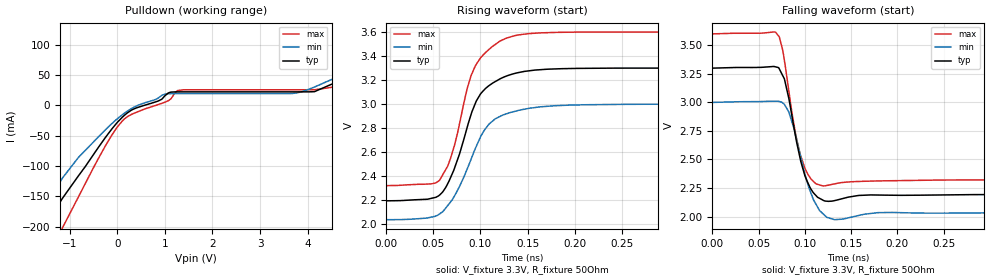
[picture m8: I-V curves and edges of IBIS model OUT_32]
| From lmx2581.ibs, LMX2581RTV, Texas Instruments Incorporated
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[Model]   OUT_32
Model_type   Open_drain
Polarity   Non-Inverting
Vmeas = 3.3
Vref = 3.3
Cref = 1pF
Rref = 50
|   typ   min   max
|   (nom PVT)   (slow PVT)   (fast PVT)
C_comp   0.269p   0.254p   0.289p
|C_comp (Hi state)   0.335p   0.327p   0.337p
|C_comp (Low state)   0.269p   0.254p   0.289p
[Voltage Range]   3.3   3   3.6
[Temperature Range]   27   125   -40
[Pullup Reference]   3.3   3   3.6
[Pulldown Reference]   0   0   0
[Power Clamp Reference]   3.3   3   3.6
[GND Clamp Reference]   0   0   0
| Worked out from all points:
|   slope of the pulldown table from 0 to 0.495 V, typ, clamps not added: 18.7 ohm
|   falling waveform, V_fixture 3.3V, R_fixture 50Ohm: 20-80 % time 16.5ps typ, 18.6ps min, 15.7ps max; typ from 3.3 V to 2.19 V
|   rising waveform, V_fixture 3.3V, R_fixture 50Ohm: 20-80 % time 29.8ps typ, 34.5ps min, 27.4ps max; typ from 2.19 V to 3.3 V
[Pulldown]
|   Voltage   I(typ)   I(min)   I(max)
-3.3V     -460.2mA   -399.9mA   -604.6mA
-2.122V   -291mA     -253.2mA   -382.1mA
-1.3V     -172.4mA   -139.2mA   -229.3mA
-1.152V   -153.4mA   -120.1mA   -202.1mA
16.5mV    -26.96mA   -21.26mA   -34.35mA
293.7mV   -8.221mA   -5.668mA   -15.28mA
986.7mV   14.45mA    18.01mA    4.661mA
1.403V    22.09mA    19.23mA    25.53mA
3.67V     22.1mA     19.42mA    25.56mA
4.145V    22.52mA    30.13mA    25.58mA
4.729V    42.4mA     50.37mA    32.14mA
6.6V      128mA      123.1mA    128.5mA
[Ramp]
R_load = 50
|   typ   min   max
dV/dt_r   0.662764/2.98253e-11   0.576799/3.45445e-11   0.766967/2.7376e-11
dV/dt_f   0.662835/1.65323e-11   0.576841/1.85913e-11   0.767074/1.56776e-11
[Falling Waveform]
V_fixture = 3.3V
V_fixture_min = 3V
V_fixture_max = 3.6V
R_fixture = 50Ohm
C_fixture = 0F
|   Time   V(typ)   V(min)   V(max)
0s        3.3V       3V         3.6V
72.27ps   3.294V     3.008V     3.574V
76.91ps   3.22V      2.99V      3.415V
82.56ps   3.037V     2.917V     3.102V
94.73ps   2.514V     2.548V     2.55V
105.5ps   2.255V     2.228V     2.342V
119.7ps   2.143V     2.023V     2.268V
132.2ps   2.14V      1.973V     2.287V
194.1ps   2.187V     2.036V     2.314V
900ps     2.195V     2.039V     2.322V
[Rising Waveform]
V_fixture = 3.3V
V_fixture_min = 3V
V_fixture_max = 3.6V
R_fixture = 50Ohm
C_fixture = 0F
|   Time   V(typ)   V(min)   V(max)
0s        2.195V     2.039V     2.322V
56.51ps   2.243V     2.086V     2.365V
68.24ps   2.388V     2.186V     2.549V
75.87ps   2.543V     2.286V     2.766V
86.1ps    2.812V     2.464V     3.135V
94.73ps   3.009V     2.633V     3.321V
109.1ps   3.154V     2.834V     3.455V
138.9ps   3.26V      2.945V     3.573V
252.3ps   3.299V     2.998V     3.6V
900ps     3.3V       3V         3.6V
